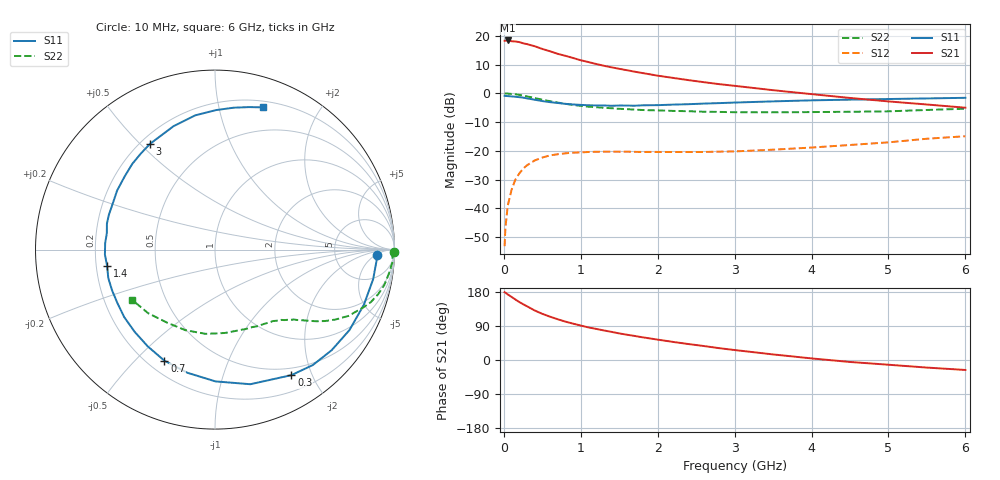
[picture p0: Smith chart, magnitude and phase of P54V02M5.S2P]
! SIEMENS Small Signal Semiconductors
! BFP183
! Si NPN RF Bipolar Junction Transistor in SOT143
! VCE = 4 V  IC = 2.5 mA
! Common Emitter S-Parameters:  March  1996
# GHz  S  MA  R  50
!  f  S11  S21  S12  S22
! GHz  MAG  ANG  MAG  ANG  MAG  ANG  MAG  ANG
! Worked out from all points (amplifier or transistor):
!   36 points, 10 MHz to 6 GHz, reference 50 ohm
!   highest |S21| = 18.4 dB at 50 MHz (marker M1)
!   |S21| within 3 dB of that: start of sweep to 506.2 MHz
!   unconditionally stable (mu >= 1): 1.982 GHz to 5.757 GHz
!   at 250 MHz: K = 0.13, MSG = 21.8 dB, |S12| = -26.2 dB
!   at 1.4 GHz: K = 0.72, MSG = 14.7 dB, |S12| = -20.3 dB
!   at 6 GHz: K = 0.96, MSG = 5.0 dB, |S12| = -14.9 dB
!   S11 on the Smith chart (normalised r, x): 10 MHz: 18, -6; 300 MHz: 0.40, -1.71; 700 MHz: 0.27, -0.61; 1.4 GHz: 0.25, -0.07; 3 GHz: 0.24, +0.54; 6 GHz: 0.26, +1.36
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0.01  0.9052 -1.9  8.229 178.8  0.0022 85.2  0.9984 -0.8
0.02  0.9016 -4.3  8.266 177.8  0.0045 89.5  0.9894 -1.6
0.05  0.8964 -10.6  8.317 173.1  0.011 85.5  0.9915 -4.0
0.15  0.8731 -30.9  7.98 159.6  0.0316 73.0  0.9639 -11.8
0.2  0.8582 -40.8  7.801 153.1  0.0404 68.1  0.9416 -15.4
0.25  0.8432 -49.7  7.426 147.2  0.0487 63.0  0.9165 -18.6
0.3  0.8187 -58.7  7.194 141.9  0.056 58.4  0.8867 -21.3
0.4  0.7754 -75.3  6.605 130.8  0.068 50.3  0.8305 -26.4
0.5  0.7343 -89.8  5.922 121.8  0.0765 43.5  0.7751 -30.2
0.6  0.7031 -102.7  5.395 114.3  0.0834 38.3  0.7308 -33.0
0.7  0.6801 -114.5  4.873 107.5  0.0873 34.1  0.6907 -35.3
0.8  0.6566 -124.8  4.496 101.3  0.0907 30.4  0.6582 -37.1
0.9  0.6405 -134.3  4.122 95.9  0.0929 27.5  0.6285 -38.8
1.1  0.6201 -151.2  3.501 86.0  0.0956 22.6  0.5868 -41.6
1.4  0.608 -171.6  2.835 74.2  0.097 17.9  0.5507 -45.5
1.8  0.6193 166.5  2.257 60.0  0.0957 15.9  0.5134 -50.8
2.2  0.637 148.9  1.857 47.7  0.0955 15.3  0.495 -57.0
3  0.6916 121.5  1.352 26.3  0.0978 19.1  0.47 -72.3
3.5  0.7253 108.6  1.135 14.7  0.1048 22.2  0.4678 -83.2
4.5  0.7773 89.6  0.832 -5.2  0.1265 24.8  0.4784 -110.1
5.5  0.8162 76.6  0.64 -20.0  0.1625 23.8  0.514 -136.4
6  0.8366 71.3  0.563 -26.3  0.1796 20.3  0.5406 -148.9
